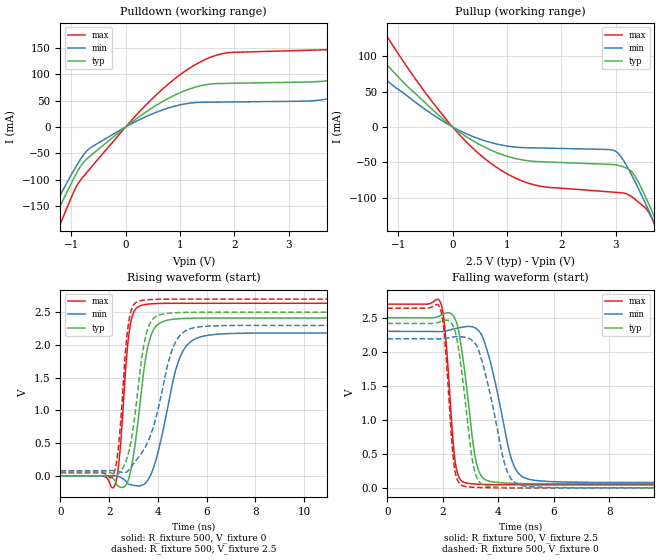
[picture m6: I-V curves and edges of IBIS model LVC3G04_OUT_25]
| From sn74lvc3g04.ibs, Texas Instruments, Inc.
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[Model]   LVC3G04_OUT_25
Model_type  Output
Vref =   0
Rref =   500
Cref =   30p
Vmeas =   1.25
| variable   typ   min   max
C_comp   9.77pF   6.16pF   14.04pF
| C_pullup   9.65pF   6.16pF   11.31pF
| C_pulldown   9.89pF   6.53pF   14.04pF
[Temperature Range]   40   100   -40
| Ambient temperature   25   85   -40
[Voltage range]   2.5   2.3   2.7
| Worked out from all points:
|   slope of the pulldown table from 0 to 0.375 V, typ, clamps not added: 13.1 ohm
|   slope of the pullup table from 0 to 0.375 V, typ, clamps not added: 19.1 ohm
|   rising waveform, R_fixture 500, V_fixture 0: 20-80 % time 499ps typ, 786ps min, 315ps max; typ from 0 V to 2.41 V
|   falling waveform, R_fixture 500, V_fixture 2.5: 20-80 % time 442ps typ, 694ps min, 283ps max; typ from 2.5 V to 0.06 V
|   rising waveform, R_fixture 500, V_fixture 2.5: 20-80 % time 527ps typ, 930ps min, 321ps max; typ from 0.06 V to 2.5 V
|   falling waveform, R_fixture 500, V_fixture 0: 20-80 % time 430ps typ, 690ps min, 272ps max; typ from 2.42 V to 0 V
[Pulldown]
| LVC3G04_OUT_25
|   Voltage   I(typ)   I(min)   I(max)
-5V       -962mA     -863.3mA   -1.124A
-1.53V    -221.1mA   -192.5mA   -267.7mA
-1.155V   -139.5mA   -119.8mA   -172mA
-665mV    -56.23mA   -40.89mA   -80.16mA
525mV     38.75mA    26.4mA     57.3mA
1.435V    79.4mA     46.8mA     126.7mA
3.83V     89.86mA    55.4mA     148.1mA
5.34V     157.5mA    105.8mA    231.8mA
5.91V     188.7mA    52.62mA    283.1mA
6.525V    93.57mA    53.13mA    299.2mA
7.5V      94.02mA    54.05mA    161.3mA
10V       98.03mA    56.54mA    166.6mA
[Pullup]
| LVC3G04_OUT_25
|   Voltage   I(typ)   I(min)   I(max)
-5V       476.9mA    373.6mA    668.8mA
-2.355V   194.1mA    148.5mA    277.6mA
-1.77V    138.1mA    104.6mA    199.1mA
-1.305V   96.51mA    72.23mA    140.3mA
-155mV    9.734mA    7.01mA     14.36mA
765mV     -34.86mA   -23.35mA   -54.93mA
1.6V      -49.31mA   -29.85mA   -83.81mA
2.995V    -53.63mA   -34.3mA    -92.61mA
3.335V    -67.41mA   -74.46mA   -101.3mA
3.72V     -128.9mA   -137.4mA   -139.3mA
3.8V      -143.3mA   -151.1mA   -154.4mA
10V       -1.404A    -1.319A    -1.567A
[Ramp]
| LVC3G04_OUT_25
| variable   typ   min   max
dV/dt_r   1.55/5.40E-10   1.40/8.44E-10   1.69/3.44E-10
dV/dt_f   1.51/4.62E-10   1.38/7.27E-10   1.64/2.95E-10
R_load = 500
[Rising Waveform]
| LVC3G04_OUT_25
R_fixture =   500
C_fixture =   0
L_fixture =   0
V_fixture =   0
V_fixture_min = 0
V_fixture_max = 0
|   Time   V(typ)   V(min)   V(max)
0s        123.6pV    5.828nV    2.514nV
2.225ns   -66.04mV   359.1uV    -149.8mV
2.42ns    -167.1mV   -16.26mV   290.9mV
2.83ns    -4.194mV   -131.4mV   2.224V
3.32ns    1.289V     -147.1mV   2.604V
3.58ns    1.962V     -68.58mV   2.623V
3.895ns   2.273V     213.7mV    2.632V
4.855ns   2.4V       1.764V     2.637V
5.765ns   2.41V      2.125V     2.637V
24.99ns   2.411V     2.183V     2.637V
[Falling Waveform]
| LVC3G04_OUT_25
R_fixture =   500
C_fixture =   0
L_fixture =   0
V_fixture =   2.5
V_fixture_min = 2.3
V_fixture_max = 2.7
|   Time   V(typ)   V(min)   V(max)
0s        2.5V       2.3V       2.7V
1.915ns   2.532V     2.296V     2.727V
2.08ns    2.563V     2.302V     2.325V
2.445ns   2.479V     2.341V     392.7mV
2.81ns    1.648V     2.367V     74.2mV
3.145ns   509mV      2.355V     56.77mV
3.375ns   183.6mV    2.265V     51.58mV
4.49ns    67.36mV    405.6mV    45.58mV
5.105ns   62.62mV    126.7mV    45.23mV
24.99ns   60.11mV    78.16mV    45.05mV
[Rising Waveform]
| LVC3G04_OUT_25
R_fixture =   500
C_fixture =   0
L_fixture =   0
V_fixture =   2.5
V_fixture_min = 2.3
V_fixture_max = 2.7
|   Time   V(typ)   V(min)   V(max)
0s        60.06mV    78.1mV     45.02mV
2.165ns   31.07mV    79.78mV    15.93mV
2.39ns    34.11mV    68.51mV    480.1mV
2.79ns    348.8mV    82.81mV    2.326V
3.215ns   1.437V     291.2mV    2.669V
3.47ns    2.088V     434.1mV    2.686V
3.77ns    2.385V     698.2mV    2.695V
4.61ns    2.49V      1.952V     2.7V
5.415ns   2.499V     2.258V     2.7V
24.99ns   2.5V       2.3V       2.7V
[Falling Waveform]
| LVC3G04_OUT_25
R_fixture =   500
C_fixture =   0
L_fixture =   0
V_fixture =   0
V_fixture_min = 0
V_fixture_max = 0
|   Time   V(typ)   V(min)   V(max)
0s        2.416V     2.191V     2.64V
1.9ns     2.442V     2.189V     2.642V
2.055ns   2.461V     2.193V     2.26V
2.415ns   2.338V     2.221V     318.4mV
2.785ns   1.369V     2.214V     22.5mV
3.055ns   437.9mV    2.17V      10.18mV
3.285ns   106.1mV    2.032V     5.654mV
4.26ns    5.94mV     316.4mV    619uV
4.825ns   2.028mV    36.78mV    235.8uV
24.99ns   40.77uV    57.53uV    30.49uV
